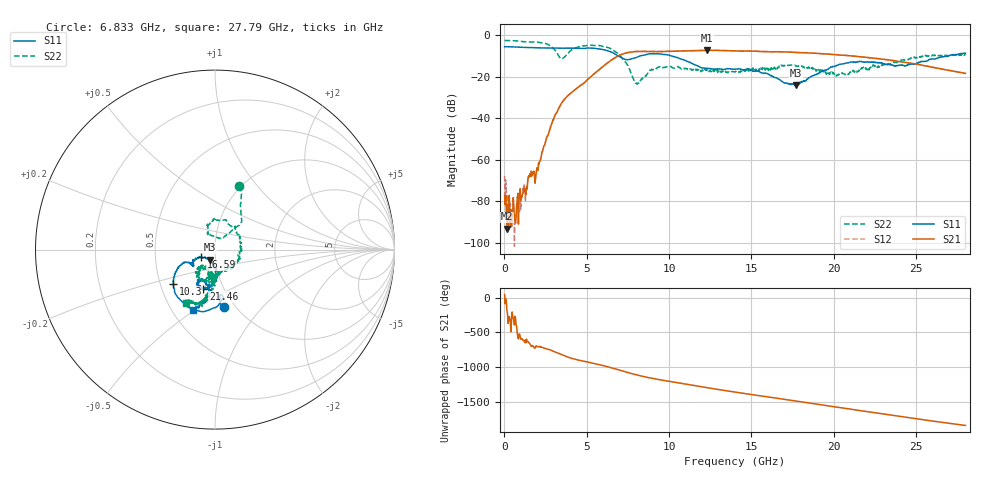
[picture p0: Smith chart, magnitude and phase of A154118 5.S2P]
!  2-Port S-parameters saved by WinCal
! VAR MeasName=S-Parameters (CALIBRATED_DATA) read from VNA (N5230A)
! VAR MeasDate=2015-9-10 14:34:49
! VAR NAME=A154118 5
! VAR FILENAME=A154118 5.S2P
! VAR DATE=2015-9-10 14:34:49
! VAR PHYS_PORTS=1,2
# Hz S DB R 50
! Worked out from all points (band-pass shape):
!   801 points, 10 MHz to 28 GHz, reference 50 ohm
!   highest |S21| = -7.37 dB at 12.29 GHz (marker M1); lowest = -93.1 dB at 149.9 MHz (marker M2)
!   |S21| within 3 dB of the highest: 6.832 GHz to 21.42 GHz (14.59 GHz wide, 103 % of centre)
!   lowest |S11| = -24.3 dB at 17.71 GHz (marker M3), VSWR 1.13, Z = 47.1 - j5.22 ohm
!   |S11| at or under -10 dB: 6.885 GHz to 8.285 GHz (1.399 GHz wide, 18.4 % of centre); 10.1 GHz to 27 GHz (16.9 GHz wide, 91.1 % of centre)
!   |S22| runs from -23.8 to -2.7 dB; largest |S21 - S12| = 0.0081
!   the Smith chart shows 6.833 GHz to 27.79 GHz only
!   S11 on the Smith chart (normalised r, x): 6.833 GHz: 0.89, -0.64; 10.3 GHz: 0.59, -0.24; 16.59 GHz: 0.85, -0.07; 21.46 GHz: 0.80, -0.37; 27.79 GHz: 0.63, -0.49
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1e7  -5.69 179.5  -77.23 43.6  -67.86 171.0  -2.66 179.8
1.4995e8  -5.66 175.1  -93.13 167.3  -84.44 164.7  -2.69 176.3
7.0975e8  -5.82 157.7  -87.31 -28.3  -86.11 -50.6  -2.85 162.5
1.9693e9  -6.18 119.4  -63.88 13.2  -64.39 15.3  -3.48 129.1
2.66905e9  -6.31 95.7  -47.69 -25.7  -47.65 -25.2  -4.67 91.1
3.193862e9  -6.31 76.1  -37.04 -72.8  -37.01 -72.7  -8.71 25.7
3.753662e9  -6.35 53.7  -29.96 -127.4  -29.96 -127.2  -9.83 -108.8
4.698325e9  -6.46 12.2  -23.90 169.5  -23.88 169.7  -5.34 166.4
5.782938e9  -6.76 -38.3  -16.56 113.8  -16.49 114.0  -5.18 119.3
6.832562e9  -9.74 -81.0  -10.37 48.1  -10.31 47.8  -8.48 69.6
8.022138e9  -10.81 -82.8  -7.96 -31.7  -7.91 -31.8  -23.16 68.8
9.351662e9  -9.09 -117.2  -8.04 -97.9  -7.94 -98.2  -15.47 93.9
1.029632e10  -10.46 -140.8  -7.83 -136.9  -7.76 -137.6  -15.98 59.0
1.229061e10  -16.04 -150.5  -7.37 145.1  -7.35 144.4  -16.61 -26.7
1.4005e10  -16.48 -145.5  -7.69 81.6  -7.67 81.0  -17.80 -78.9
1.659408e10  -21.02 -151.6  -8.10 -8.6  -8.05 -9.1  -15.50 -104.5
1.771368e10  -24.26 -115.8  -8.42 -48.4  -8.42 -48.6  -15.04 -119.9
1.869332e10  -19.68 -88.7  -8.73 -82.4  -8.74 -82.7  -15.68 -125.1
2.145734e10  -12.80 -106.7  -10.38 -179.2  -10.30 -180.0  -17.73 -103.8
2.334666e10  -14.12 -116.8  -12.03 114.7  -11.98 113.8  -14.24 -92.0
2.779008e10  -8.91 -110.3  -18.17 -32.2  -18.18 -33.1  -9.40 -118.5
2.8e10  -8.81 -111.4  -18.51 -38.5  -18.51 -39.6  -9.25 -119.5
